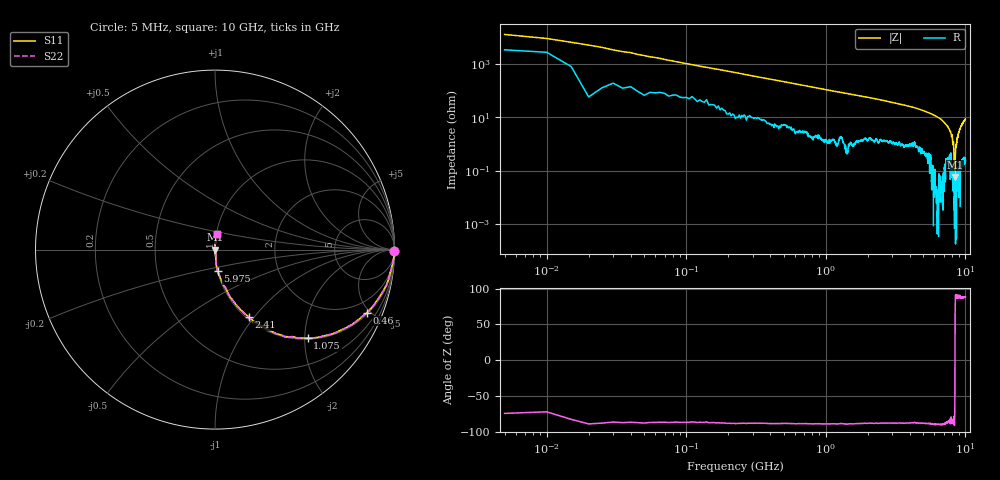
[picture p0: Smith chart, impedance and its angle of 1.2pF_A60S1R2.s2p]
! Amotech Co.,Ltd.
! http://www.amotech.co.kr/
! Part Number: A60S1R2
! These Parameters are Measured in Series Mode Connection
! Operation Temp=25[degC], DC Bias Voltage=0[V]
! Freq. Start=5[MHz] Stop=10[GHz], 2000[Steps]
! Date: Monday, July 13, 2020, 01:49:07
# GHZ S RI R 50.000000
!Freq.(Hz) S11(Real) S11(Imag) S21(Real) S21(Imag) S12(Real) S12(Imag) S22(Real) S22(Imag)
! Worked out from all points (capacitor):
!   2000 points, 5 MHz to 10 GHz, reference 50 ohm
!   read as one part in series: C = 1.5 pF near 55 MHz
!   lowest |Z| = 57.6 mohm at 8.415 GHz (marker M1)
!   series resonance near 8.417 GHz, so ESL is about 240 pH
!   S11 on the Smith chart (normalised r, x): 5 MHz: open; 460 MHz: 1.08, -4.80; 1.075 GHz: 1.02, -2.07; 2.41 GHz: 1.02, -0.94; 5.975 GHz: 1.00, -0.24; 10 GHz: 1.00, +0.18
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0.005  0.998 -0.00725  0.00205 0.00725  0.00205 0.00725  0.998 -0.00725
0.075  0.992 -0.0698  0.00804 0.0698  0.00804 0.0698  0.992 -0.0698
0.14  0.9759 -0.1257  0.0241 0.1257  0.0241 0.1257  0.9759 -0.1257
0.46  0.8485 -0.3508  0.1515 0.3508  0.1515 0.3508  0.8485 -0.3508
1.075  0.5165 -0.4943  0.4835 0.4943  0.4835 0.4943  0.5165 -0.4943
1.675  0.3172 -0.4562  0.6828 0.4562  0.6828 0.4562  0.3172 -0.4562
2.41  0.1867 -0.3771  0.8133 0.3771  0.8133 0.3771  0.1867 -0.3771
3.34  0.1023 -0.2854  0.8977 0.2854  0.8977 0.2854  0.1023 -0.2854
5.005  0.0357 -0.1716  0.9643 0.1716  0.9643 0.1716  0.0357 -0.1716
5.975  0.014 -0.1192  0.986 0.1192  0.986 0.1192  0.014 -0.1192
6.67  0.00727 -0.0855  0.9927 0.0855  0.9927 0.0855  0.00727 -0.0855
7.47  0.00448 -0.0452  0.9955 0.0452  0.9955 0.0452  0.00448 -0.0452
8.025  0.00116 -0.0217  0.9988 0.0217  0.9988 0.0217  0.00116 -0.0217
8.125  0.000817 -0.0103  0.9992 0.0103  0.9992 0.0103  0.000817 -0.0103
8.23  0.000677 -0.0113  0.9993 0.0113  0.9993 0.0113  0.000677 -0.0113
8.335  1.98e-05 -0.000972  1 0.000972  1 0.000972  1.98e-05 -0.000972
8.375  0.000193 -0.00136  0.9998 0.00136  0.9998 0.00136  0.000193 -0.00136
8.415  0.00057 -8.44e-05  0.9994 8.44e-05  0.9994 8.44e-05  0.00057 -8.44e-05
8.525  0.0002 0.00726  0.9998 -0.00726  0.9998 -0.00726  0.0002 0.00726
8.74  0.000894 0.0163  0.9991 -0.0163  0.9991 -0.0163  0.000894 0.0163
9.115  0.00232 0.0355  0.9977 -0.0355  0.9977 -0.0355  0.00232 0.0355
10  0.01 0.087  0.99 -0.087  0.99 -0.087  0.01 0.087
